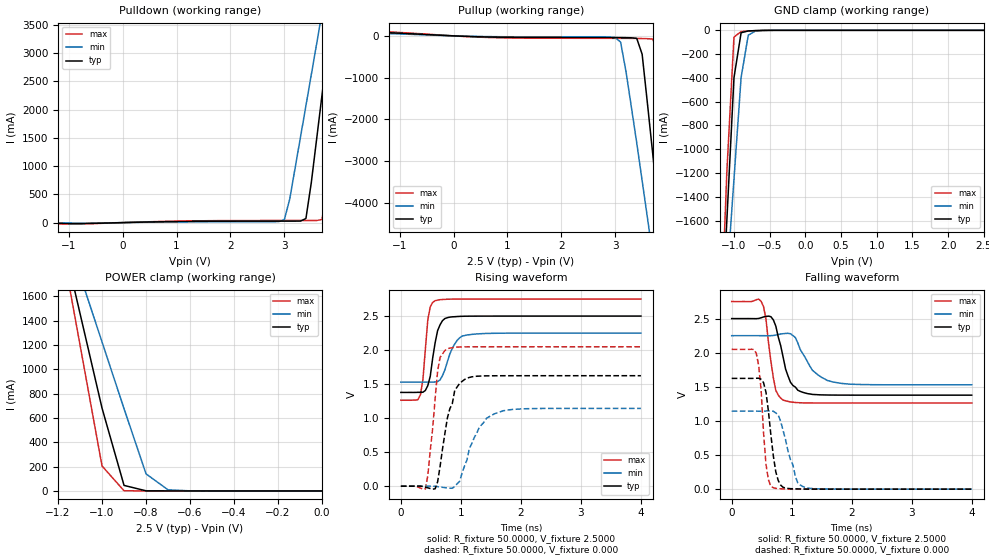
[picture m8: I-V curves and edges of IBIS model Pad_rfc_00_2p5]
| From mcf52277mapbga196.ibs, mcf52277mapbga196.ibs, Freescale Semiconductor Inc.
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|   Model Pad_rfc_00
[Model]   Pad_rfc_00_2p5
Model_type   3-state
Polarity   Non-Inverting
Enable   Active-High
Vmeas =   1.2500V
C_comp   1.7450pF   1.6200pF   1.8900pF
[Temperature Range]   25.0000   0.1500k   -40.0000
[Voltage Range]   2.5000V   2.2500V   2.7500V
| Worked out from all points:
|   slope of the pulldown table from 0 to 0.375 V, typ, clamps not added: 43.3 ohm
|   slope of the pullup table from 0 to 0.375 V, typ, clamps not added: 20.6 ohm
|   GND clamp passes 1 mA (typ) near -0.62 V on its own axis
|   POWER clamp passes 1 mA (typ) near -0.80 V on its own axis
|   rising waveform, R_fixture 50.0000, V_fixture 2.5000: 20-80 % time 124ps typ, 193ps min, 84.2ps max; typ from 1.38 V to 2.5 V
|   rising waveform, R_fixture 50.0000, V_fixture 0.000: 20-80 % time 216ps typ, 324ps min, 130ps max; typ from 0 V to 1.62 V
|   falling waveform, R_fixture 50.0000, V_fixture 2.5000: 20-80 % time 199ps typ, 323ps min, 134ps max; typ from 2.5 V to 1.38 V
|   falling waveform, R_fixture 50.0000, V_fixture 0.000: 20-80 % time 133ps typ, 211ps min, 98.1ps max; typ from 1.62 V to 0 V
[Pulldown]
| voltage   I(typ)   I(min)   I(max)
-2.5V     -560uA     -370uA     -680uA
-900mV    -18.6mA    -9.254mA   -24.67mA
3V        26.19mA    51.53mA    37.09mA
3.1V      26.26mA    418.4mA    37.18mA
3.4V      71.84mA    2.066A     37.42mA
3.5V      707.5mA    2.616A     37.51mA
3.6V      1.486A     3.167A     37.7mA
3.7V      2.266A     3.719A     54.77mA
3.8V      3.046A     4.271A     740.6mA
4V        4.609A     5.375A     2.733A
4.2V      6.175A     6.481A     4.73A
5V        12.45A     10.91A     12.74A
[Pullup]
| voltage   I(typ)   I(min)   I(max)
-2.5V     111mA      87.16mA    137.7mA
3V        -40.88mA   -41.78mA   -59.42mA
3.1V      -41.63mA   -148.6mA   -59.58mA
3.2V      -43.38mA   -851.7mA   -59.75mA
3.4V      -61.51mA   -2.572A    -61.63mA
3.5V      -440.3mA   -3.477A    -64.43mA
3.6V      -1.643A    -4.384A    -68.14mA
3.7V      -2.874A    -5.29A     -76.87mA
3.8V      -4.121A    -6.198A    -491mA
4V        -6.635A    -8.024A    -3.585A
4.2V      -9.165A    -9.859A    -6.704A
5V        -19.32A    -17.25A    -19.34A
[GND_clamp]
| voltage   I(typ)   I(min)   I(max)
-2.5V     -19.27A    -14.9A     -23.25A
-1.2V     -2.833A    -2.997A    -2.746A
-1.1V     -1.601A    -2.108A    -1.195A
-1V       -399mA     -1.252A    -56.61mA
-900mV    -20.31mA   -398.2mA   -10.19mA
-800mV    -5.193mA   -41.09mA   -5.939mA
-700mV    -2.389mA   -6.145mA   -2.797mA
-400mV    -10.19uA   -60.07uA   -3.537uA
2.5V      1.128nA    208.6nA    39.38pA
[POWER_clamp]
| voltage   I(typ)   I(min)   I(max)
-2.5V     12.42A     9.511A     15.21A
-1.2V     2.239A     2.325A     2.196A
-1.1V     1.46A      1.775A     1.201A
-1V       681mA      1.225A     205.3mA
-900mV    45.39mA    676.7mA    1.42mA
-800mV    926.4uA    140.3mA    9.917uA
-700mV    19.11uA    9.036mA    78.78nA
-600mV    428.3nA    583.1uA    762.2pA
0V        1.128nA    78.54nA    61.1pA
[Ramp]
| variable   typ   min   max
dV/dt_r   0.9742/0.2017n   0.6859/0.3273n   1.2294/0.1304n
dV/dt_f   0.6732/0.2045n   0.4323/0.3206n   0.8921/0.1350n
R_load = 50.0000
[Rising Waveform]
R_fixture = 50.0000
V_fixture = 2.5000
V_fixture_min = 2.2500
V_fixture_max = 2.7500
| time   V(typ)   V(min)   V(max)
0s        1.378V     1.53V      1.263V
326.5ps   1.38V      1.529V     1.345V
367.3ps   1.381V     1.53V      1.564V
449ps     1.478V     1.53V      2.444V
489.8ps   1.615V     1.53V      2.636V
571.4ps   2.11V      1.532V     2.726V
693.9ps   2.433V     1.625V     2.744V
857.1ps   2.489V     2.026V     2.749V
1.02ns    2.497V     2.207V     2.75V
4ns       2.5V       2.25V      2.75V
[Rising Waveform]
R_fixture = 50.0000
V_fixture = 0.000
| time   V(typ)   V(min)   V(max)
0s        305.8pV    1.949nV    177.1pV
408.2ps   -15.01mV   402uV      -42.58mV
449ps     -23.72mV   900.2uV    155.4mV
612.2ps   63.33mV    -6.445mV   1.689V
653.1ps   287.7mV    -12.39mV   1.892V
775.5ps   1.004V     -26.09mV   2.021V
979.6ps   1.51V      70.94mV    2.046V
1.306ns   1.618V     862.9mV    2.049V
1.551ns   1.623V     1.061V     2.049V
4ns       1.624V     1.143V     2.049V
[Falling Waveform]
R_fixture = 50.0000
V_fixture = 2.5000
V_fixture_min = 2.2500
V_fixture_max = 2.7500
| time   V(typ)   V(min)   V(max)
0s        2.5V       2.25V      2.75V
489.8ps   2.512V     2.25V      2.754V
571.4ps   2.532V     2.249V     2.49V
734.7ps   2.391V     2.258V     1.449V
857.1ps   1.934V     2.279V     1.306V
979.6ps   1.567V     2.278V     1.279V
1.102ns   1.45V      2.142V     1.268V
1.347ns   1.388V     1.74V      1.264V
1.674ns   1.379V     1.574V     1.263V
4ns       1.378V     1.53V      1.263V
[Falling Waveform]
R_fixture = 50.0000
V_fixture = 0.000
| time   V(typ)   V(min)   V(max)
0s        1.624V     1.143V     2.049V
408.2ps   1.626V     1.143V     1.995V
489.8ps   1.611V     1.143V     1.457V
530.6ps   1.561V     1.143V     829.8mV
571.4ps   1.42V      1.145V     362.6mV
653.1ps   793.8mV    1.148V     38.91mV
816.3ps   59.04mV    994.3mV    5.328mV
1.061ns   4.378mV    186.2mV    595.2uV
1.225ns   1.343mV    25.01mV    56.29uV
4ns       1.921uV    1.828uV    2.056uV
